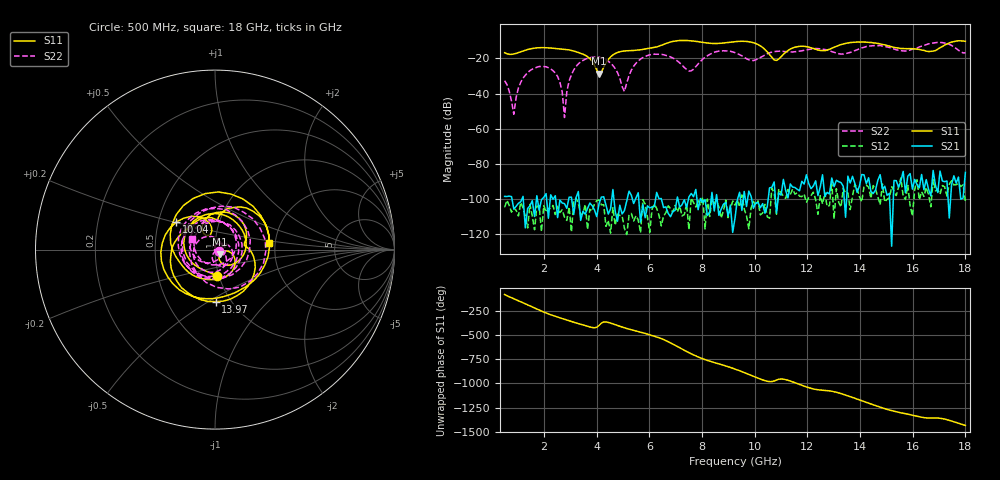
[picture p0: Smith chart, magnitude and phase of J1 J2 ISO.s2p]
!Agilent Technologies,N5230A,MY45001360,A.07.50.67
!Agilent N5230A: A.07.50.67
!Date: Tuesday, April 16, 2024 16:22:33
!Correction: S11(Full 2 Port(1,2))
!S21(Full 2 Port(1,2))
!S12(Full 2 Port(1,2))
!S22(Full 2 Port(1,2))
!S2P File: Measurements: S11, S21, S12, S22:
# Hz S  dB  R 50
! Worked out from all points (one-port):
!   201 points, 500 MHz to 18 GHz, reference 50 ohm
!   lowest |S11| = -28.7 dB at 4.088 GHz (marker M1), VSWR 1.08, Z = 52.7 - j2.65 ohm
!   |S11| at or under -10 dB: start of sweep to 7.056 GHz; 7.542 GHz to end of sweep
!   S11 on the Smith chart (normalised r, x): 500 MHz: 0.98, -0.29; 10.04 GHz: 0.62, +0.21; 13.97 GHz: 0.85, -0.54; 18 GHz: 1.86, +0.16
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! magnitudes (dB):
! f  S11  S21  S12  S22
! 500 MHz  -16.8  -98.4  -104.6  -32.7
! 850 MHz  -17.5  -105.6  -105.0  -51.8
! 1.025 GHz  -16.7  -102.3  -109.5  -36.8
! 1.288 GHz  -15.4  -116.2  -109.7  -29.6
! 2.25 GHz  -14.1  -97.5  -105.3  -26.0
! 2.6 GHz  -14.6  -100.4  -107.6  -33.6
! 2.775 GHz  -14.9  -102.5  -110.1  -53.6
! 2.95 GHz  -15.2  -98.8  -104.4  -32.8
! 3.475 GHz  -17.6  -106.8  -108.1  -21.2
! 4.088 GHz  -28.7  -102.5  -100.4  -19.4
! 4.612 GHz  -18.0  -94.5  -104.8  -24.0
! 5.05 GHz  -15.8  -106.4  -116.4  -38.8
! 5.487 GHz  -15.4  -99.4  -109.4  -22.8
! 6.362 GHz  -13.1  -99.7  -108.9  -17.6
! 7.5 GHz  -10.0  -98.7  -117.3  -27.2
! 9.25 GHz  -10.5  -110.7  -103.4  -16.8
! 10.04 GHz  -11.6  -102.1  -103.7  -20.9
! 10.82 GHz  -21.2  -107.8  -108.5  -16.0
! 12.22 GHz  -14.4  -92.5  -96.0  -14.5
! 13.97 GHz  -10.8  -92.6  -98.5  -14.6
! 15.11 GHz  -13.0  -96.7  -99.3  -13.8
! 18 GHz  -10.3  -84.7  -101.1  -16.9
